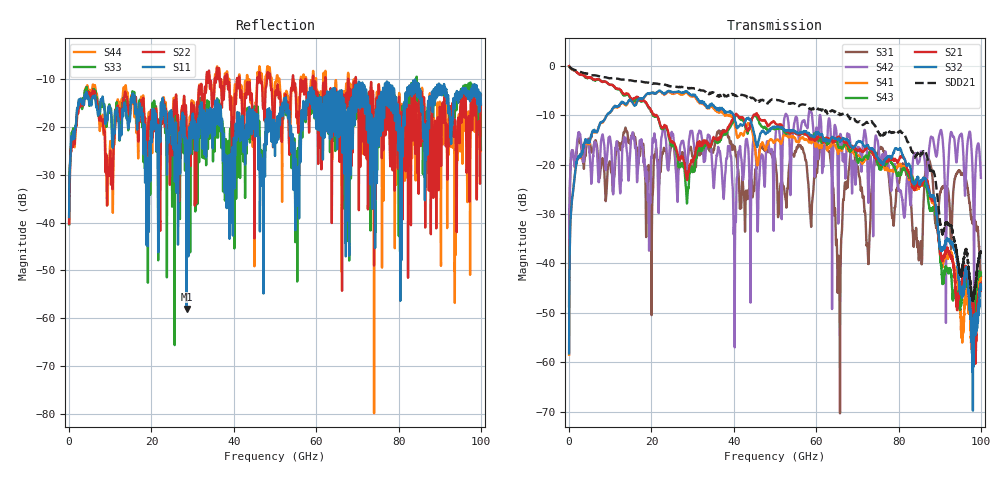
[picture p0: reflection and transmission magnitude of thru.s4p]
!Keysight Technologies,N5242B,US61255209,A.15.75.22
!Date: Tuesday, January 14, 2025 10:19:41
!Correction: S11(C  4-Port  )
!S12(C  4-Port  )
!S13(C  4-Port  )
!S14(C  4-Port  )
!S21(C  4-Port  )
!S22(C  4-Port  )
!S23(C  4-Port  )
!S24(C  4-Port  )
!S31(C  4-Port  )
!S32(C  4-Port  )
!S33(C  4-Port  )
!S34(C  4-Port  )
!S41(C  4-Port  )
!S42(C  4-Port  )
!S43(C  4-Port  )
!S44(C  4-Port  )
!S4P File: Measurements: <S11,S12,S13,S14>,
!<S21,S22,S23,S24>,
!<S31,S32,S33,S34>,
!<S41,S42,S43,S44>:
! Port[1] =
! Port[2] =
! Port[3] =
! Port[4] =
# Hz S RI R 50
! freq  S11re  S11im  S12re  S12im  S13re  S13im  S14re  S14im
!  S21re  S21im  S22re  S22im  S23re  S23im  S24re  S24im
!  S31re  S31im  S32re  S32im  S33re  S33im  S34re  S34im
!  S41re  S41im  S42re  S42im  S43re  S43im  S44re  S44im
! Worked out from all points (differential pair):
!   10000 points, 10 MHz to 100 GHz, reference 50 ohm
!   strongest paths, dB at 10 MHz, 25.01 GHz, 50.01 GHz, 75.01 GHz, 100 GHz:
!     S32: -58.2, -5.3, -12.4, -18.7, -45.0
!     S21: -0.1, -15.4, -11.5, -18.7, -45.2
!     S43: -0.1, -15.9, -12.8, -20.1, -41.9
!     S41: -58.5, -5.6, -15.3, -20.0, -42.7
!     S42: -48.6, -13.8, -16.1, -15.5, -22.7
!     S31: -48.7, -15.4, -18.6, -17.7, -42.7
!   taken as a pair (ports 1,3 in; 2,4 out), SDD21 dB: -0.1, -4.1, -6.9, -13.4, -37.7
!   lowest |S11| = -58.0 dB at 28.54 GHz (marker M1), VSWR 1.00, Z = 49.9 + j0.0743 ohm
!   |S11| at or under -10 dB: start of sweep to end of sweep
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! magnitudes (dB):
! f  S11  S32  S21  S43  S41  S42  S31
! 10 MHz  -38.9  -58.2  -0.1  -0.1  -58.5  -48.6  -48.7
! 3.92 GHz  -13.5  -15.1  -2.1  -2.2  -15.2  -16.3  -18.0
! 28.54 GHz  -58.0  -5.2  -22.5  -26.4  -5.4  -21.2  -20.9
! 62.33 GHz  -13.9  -15.0  -14.8  -15.2  -15.6  -14.8  -16.3
! 65.53 GHz  -22.1  -14.7  -14.3  -16.5  -17.1  -20.5  -39.6
! 80.97 GHz  -22.6  -18.0  -18.3  -21.0  -20.4  -27.3  -19.8
! 100 GHz  -15.4  -45.0  -45.2  -41.9  -42.7  -22.7  -42.7
